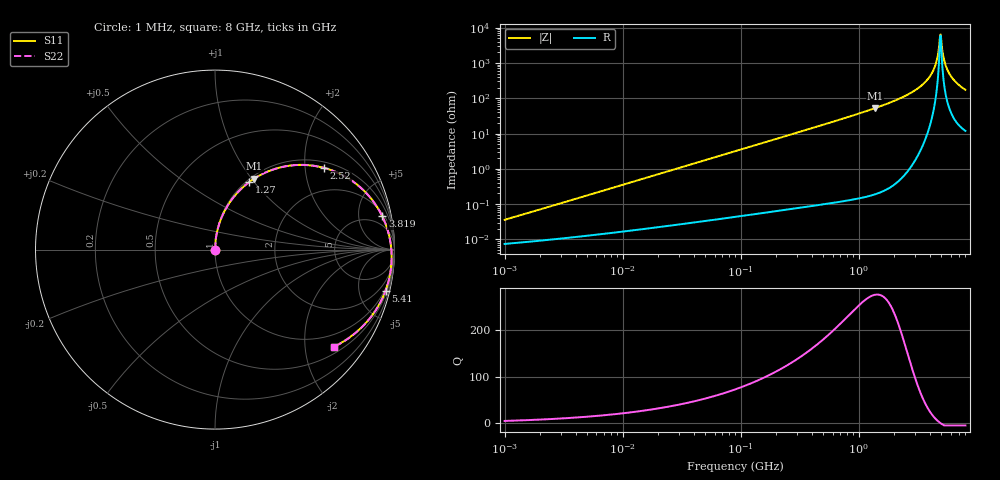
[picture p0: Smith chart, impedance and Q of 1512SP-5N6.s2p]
# MHz  S  MA  R  50
!Freq  MagS11  AngS11  MagS21  AngS21  MagS12  AngS12  MagS22  AngS22
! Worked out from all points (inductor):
!   801 points, 1 MHz to 8 GHz, reference 50 ohm
!   read as one part in series: L = 5.59 nH near 1.046 MHz
!   highest Q = 276 at 1.374 GHz (marker M1), where L = 6.07 nH
!   self-resonance near 4.89 GHz
!   S11 on the Smith chart (normalised r, x): 1 MHz: 1.00, +0.00; 1.27 GHz: 1.03, +0.94; 2.52 GHz: 1.17, +2.52; 3.819 GHz: 2.46, +9.45; 5.41 GHz: 0.81, -8.34; 8 GHz: 0.66, -2.66
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1  0.0003479 77.6  0.9999 -0.0  0.9999 -0.0  0.0003479 77.6
4.507347  0.001537 85.3  0.9999 -0.1  0.9999 -0.1  0.001537 85.3
20.08917  0.00683 87.7  0.9998 -0.4  0.9998 -0.4  0.00683 87.7
89.53707  0.03042 87.3  0.9991 -1.9  0.9991 -1.9  0.03042 87.3
403.5746  0.1367 81.2  0.9897 -8.4  0.9897 -8.4  0.1367 81.2
783.1488  0.2634 73.4  0.9635 -16.3  0.9635 -16.3  0.2634 73.4
1269.652  0.42 63.3  0.906 -26.5  0.906 -26.5  0.4199 63.3
1373.551  0.4522 61.1  0.8903 -28.7  0.8903 -28.7  0.4521 61.1
1798.725  0.5776 52.1  0.8141 -37.7  0.8141 -37.7  0.5775 52.1
2519.794  0.7587 36.9  0.6467 -52.7  0.6467 -52.7  0.7586 36.9
3190.4  0.8805 23.3  0.4627 -66.0  0.4627 -66.0  0.8804 23.3
3818.786  0.9502 11.3  0.2843 -76.9  0.2843 -76.9  0.9501 11.3
4131.287  0.9701 5.8  0.1984 -81.3  0.1984 -81.3  0.97 5.8
4370.04  0.9795 1.8  0.1355 -83.4  0.1355 -83.4  0.9795 1.8
4570.939  0.9841 -1.4  0.08481 -83.1  0.08481 -83.1  0.9841 -1.4
4781.074  0.986 -4.7  0.03539 -72.3  0.03539 -72.3  0.986 -4.7
4889.737  0.9859 -6.3  0.01579 -33.6  0.01579 -33.6  0.9859 -6.3
5057.379  0.9845 -8.7  0.03423 55.4  0.03423 55.4  0.9846 -8.7
5410.103  0.9775 -13.6  0.1069 67.4  0.1069 67.4  0.9776 -13.6
5722.761  0.9675 -17.5  0.1668 66.1  0.1668 66.1  0.9677 -17.5
6261.028  0.9448 -23.7  0.2578 61.6  0.2578 61.6  0.9451 -23.7
8000  0.8559 -39.2  0.4636 47.1  0.4636 47.1  0.8567 -39.2
